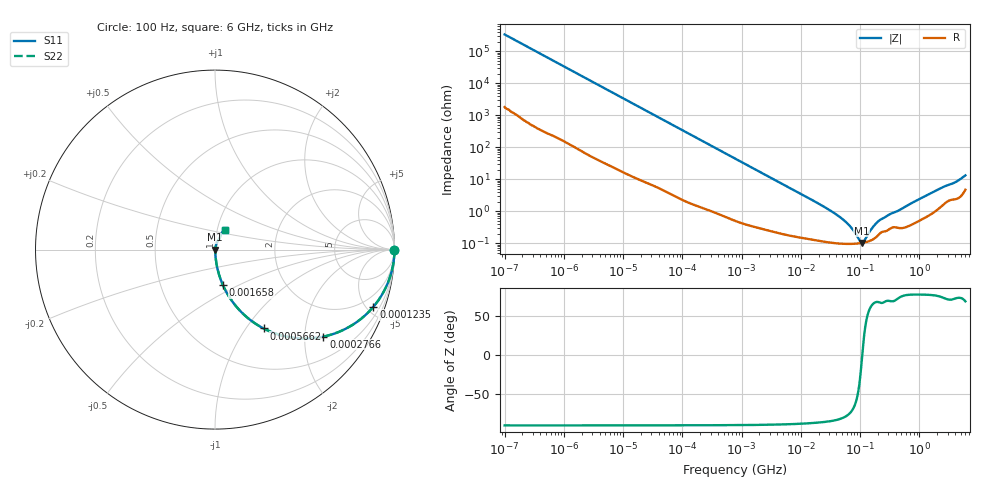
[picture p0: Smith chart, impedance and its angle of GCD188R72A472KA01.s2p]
!Murata Part Number: GCD188R72A472KA01
!These Parameters are Measured in Series Mode Connection
!Data Generated on Jan 08, 2026
!  o--ll--o
!Port1  Port2
!  o------o
!Operation Temp=25[degC], DC Bias Voltage=0[V]
!Freq. Start=100[Hz] Stop=6[GHz] 401[Steps]
# Hz S RI R 50
!Freq.(Hz) S11(Real) S11(Imag) S21(Real) S21(Imag) S12(Real) S12(Imag) S22(Real) S22(Imag)
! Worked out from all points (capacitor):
!   401 points, 100 Hz to 6 GHz, reference 50 ohm
!   read as one part in series: C = 4.76 nF near 109 Hz
!   lowest |Z| = 102 mohm at 106.7 MHz (marker M1)
!   series resonance near 108.8 MHz, so ESL is about 450 pH
!   S11 on the Smith chart (normalised r, x): 100 Hz: open; 123.5 kHz: 1.04, -5.52; 276.6 kHz: 1.02, -2.47; 566.2 kHz: 1.01, -1.21; 1.658 MHz: 1.01, -0.42; 6 GHz: 1.09, +0.25
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100  1 -0.0003  1.7e-06 0.0003  1.7e-06 0.0003  1 -0.0003
2008  0.9999 -0.00597  6.21e-05 0.00597  6.21e-05 0.00597  0.9999 -0.00597
12592  0.9984 -0.0372  0.00157 0.0372  0.00157 0.0372  0.9984 -0.0372
40335  0.9854 -0.117  0.0146 0.117  0.0146 0.117  0.9854 -0.117
123542  0.8822 -0.3189  0.1178 0.3189  0.1178 0.3189  0.8822 -0.3189
276587  0.6038 -0.4848  0.3962 0.4848  0.3962 0.4848  0.6038 -0.4848
566185  0.2711 -0.4394  0.7289 0.4394  0.7289 0.4394  0.2711 -0.4394
774597  0.1675 -0.3679  0.8325 0.3679  0.8325 0.3679  0.1675 -0.3679
1658239  0.0444 -0.1984  0.9556 0.1984  0.9556 0.1984  0.0444 -0.1984
4246196  0.00867 -0.081  0.9913 0.081  0.9913 0.081  0.00867 -0.081
1.555665e7  0.00178 -0.0222  0.9982 0.0222  0.9982 0.0222  0.00178 -0.0222
3.184506e7  0.00114 -0.0103  0.9989 0.0103  0.9989 0.0103  0.00114 -0.0103
5.211241e7  0.000983 -0.00532  0.999 0.00532  0.999 0.00532  0.000983 -0.00532
7.129496e7  0.000958 -0.00289  0.999 0.00289  0.999 0.00289  0.000958 -0.00289
9.753859e7  0.00099 -0.000728  0.999 0.000728  0.999 0.000728  0.00099 -0.000728
1.066761e8  0.00101 -0.00013  0.999 0.00013  0.999 0.00013  0.00101 -0.00013
1.166697e8  0.00104 0.00047  0.999 -0.00047  0.999 -0.00047  0.00104 0.00047
1.526266e8  0.00122 0.00233  0.9988 -0.00233  0.9988 -0.00233  0.00122 0.00233
1.909225e8  0.00161 0.00402  0.9984 -0.00402  0.9984 -0.00402  0.00161 0.00402
3.124326e8  0.00278 0.00738  0.9972 -0.00738  0.9972 -0.00738  0.00278 0.00738
4.009986e9  0.0283 0.0721  0.9717 -0.0721  0.9717 -0.0721  0.0283 0.0721
6e9  0.0577 0.1109  0.9423 -0.1109  0.9423 -0.1109  0.0577 0.1109
